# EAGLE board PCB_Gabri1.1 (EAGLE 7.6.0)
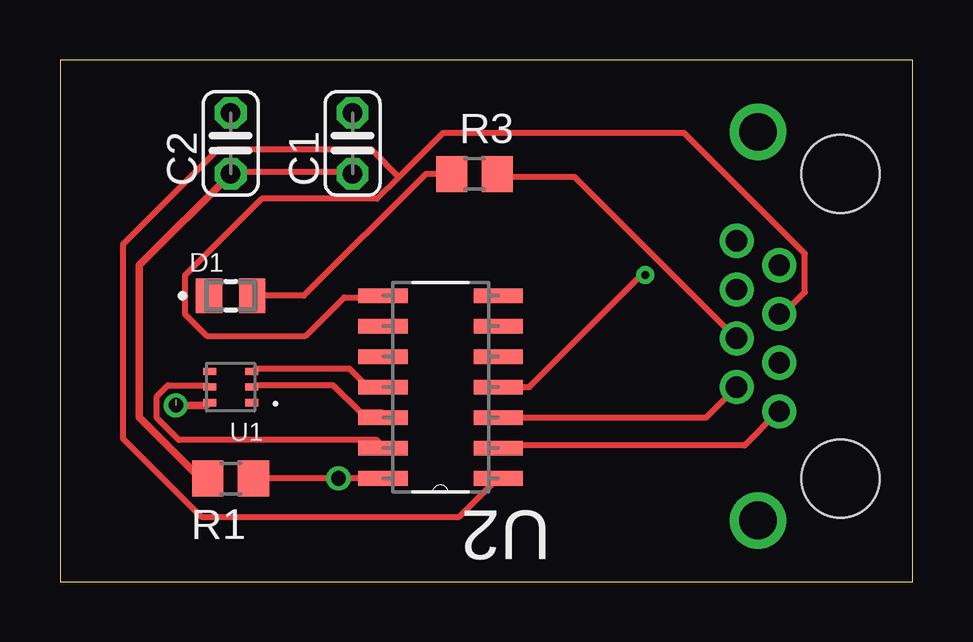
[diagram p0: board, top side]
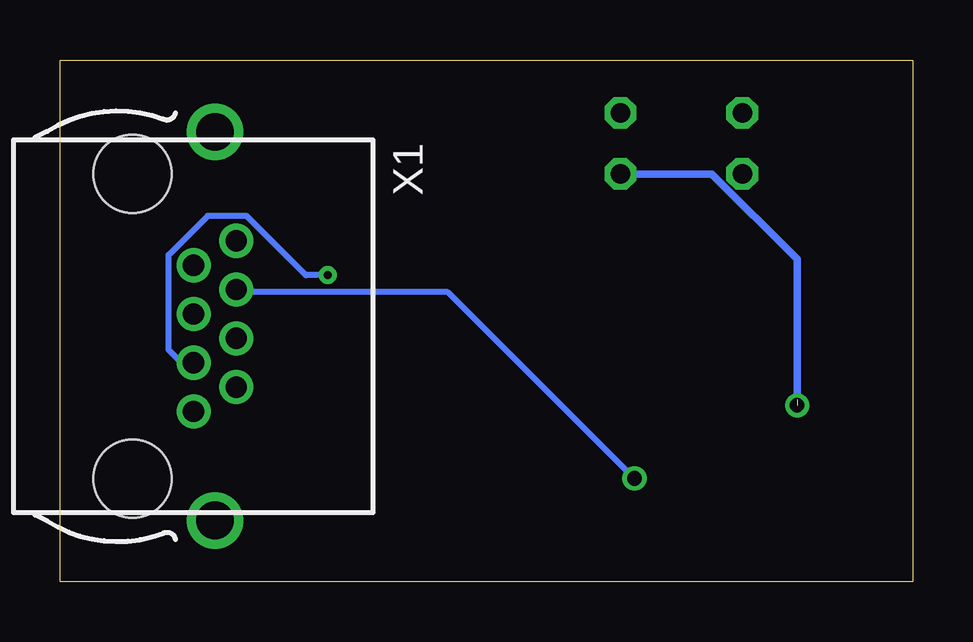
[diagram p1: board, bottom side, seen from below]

Size 35.54 x 21.77 mm. Coordinates in mm from the lower left corner, seen from the top.
Outline: 0,0 35.54,0 35.54,21.77 0,21.77 0,0
Copper layers (1*16): Top 0.035mm / dielectric 1.5mm / Bottom 0.035mm
Design rules "default": minimum track width 10mil, minimum drill 24mil, track to track 8mil, track to pad 8mil, pad to pad 8mil, via to via 8mil, smd to smd 8mil, copper to edge 40mil, drill to drill 8mil, minimum pad ring 10mil, minimum via ring 8mil, stop-mask expansion 4mil, vias tented up to drill 0mil, thermal gap 10mil
tRestrict: area 14,4.1 to 17.5,12.2; 8 lines

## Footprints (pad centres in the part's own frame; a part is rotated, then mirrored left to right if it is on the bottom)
C025-024X044 = drill 0.813 octagon: 1 -1.27,0; 2 1.27,0
LEDC2012X70N = smd 1.1 x 1.45: A 0.9,0; C -0.9,0
R0805 = smd 1.3 x 1.5: 1 -0.95,0; 2 0.95,0
VISHAY_VEML6030_2X2X0.87 = smd 0.55 x 0.3: 1 -0.875,0.65; 2 -0.875,0; 3 -0.875,-0.65; 4 0.875,-0.65; 5 0.875,0; 6 0.875,0.65
SOIC127P600X175-14N = smd 2.057 x 0.61: 1 -4.801,7.62; 2 -4.801,6.35; 3 -4.801,5.08; 4 -4.801,3.81; 5 -4.801,2.54; 6 -4.801,1.27; 7 -4.801,0; 8 0,0; 9 0,1.27; 10 0,2.54; 11 0,3.81; 12 0,5.08; 13 0,6.35; 14 0,7.62
0446200002 = drill 0.889 pad 1.422: 1 3.556,2.54; 2 2.54,4.318; 3 1.524,2.54; 4 0.508,4.318; 5 -0.508,2.54; 6 -1.524,4.318; 7 -2.54,2.54; 8 -3.556,4.318 | drill 1.575 pad 2.286: S@1 -8.103,3.429; S@2 8.103,3.429 | hole 3.251: 6.35,0; -6.35,0

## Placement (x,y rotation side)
C1  [C025-024X044]  12.19,18.29 90 top
C2  [C025-024X044]  7.11,18.29 90 top
D1  5988170107F  [LEDC2012X70N]  7.11,11.94 0 top
R1  [R0805]  7.11,4.32 180 top
R3  [R0805]  17.27,17.02 0 top
U1  VEML6030  [VISHAY_VEML6030_2X2X0.87]  7.11,8.13 180 top
U2  TXS0104ED  [SOIC127P600X175-14N]  13.46,11.94 180 top
X1  0446200002  [0446200002]  32.51,10.67 270 bottom

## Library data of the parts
C1 C2 R1 R3 = resistor
D1 = 5988170107F; AVAILABILITY: Unavailable; DESCRIPTION: LED GREEN CLEAR 0805 SMD; MF: Dialight; MP: 5988170107F; PACKAGE: 0805 Dialight; PRICE: None
U1 = VEML6030; AVAILABILITY: Unavailable; DESCRIPTION: VEML6030 Series 2 x 2 x 0.85 mm 50 mW I2C High Accuracy Ambient Light Sensor; MF: Vishay; MP: VEML6030; PACKAGE: SMD-6 Vishay; PRICE: None
U2 = TXS0104ED; AVAILABILITY: Unavailable; DESCRIPTION: 4-Bit Bidirectional Voltage-Level Shifter for Open-Drain and Push-Pull Applications 14-SOIC -40 to 85; MF: Texas Instruments; MP: TXS0104ED; PACKAGE: SOIC-14 Texas Instruments; PRICE: None
X1 = 0446200002; AVAILABILITY: Unavailable; DESCRIPTION: Conn RJ-45 RCP 8 POS 2.04mm Solder RA Thru-Hole 8 Terminal 1 Port Tray Cat 3; MF: Molex, LLC; MP: 0446200002; PACKAGE: None; PRICE: None

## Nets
A1: U2.2 X1.1
A2: U2.3 X1.2
A3: U2.4 X1.3
GND: U1.1
INT: U1.3 U2.11
LED_1: R3.2 X1.4
LED_2: D1.A R3.1
LS_VDD: C1.1 C2.1
N$1: R1.2
S$1: U1.6
SCL: U1.5 U2.13
SDA: U1.2 U2.12
VCCA: U2.1 U2.8 X1.5
VCCB: R1.1 U2.14 X1.6

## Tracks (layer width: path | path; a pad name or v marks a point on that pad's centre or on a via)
A1
  Top 0.254: U2.2 18.47,5.69 28.52,5.69 29.9,7.06 X1.1
A2
  Top 0.254: U2.3 26.92,6.86 X1.2
A3  (via drill 0.35)
  Top 0.254: U2.4 19.56,8.13 24.23,12.8 v24.38,12.8
  Bottom 0.254: X1.3 30.48,9.14 31.01,9.68 31.01,13.64 29.39,15.26 27.76,15.26 25.3,12.8 v24.38,12.8
INT
  Top 0.254: U1.3 8.18,8.89 12.06,8.89 12.75,8.2 13.44,8.2 U2.11
LED_1
  Top 0.254: R3.2 18.24,16.89 21.44,16.89 28.07,10.26 X1.4
LED_2
  Top 0.254: R3.1 15.24,17.02 10.16,11.94 D1.A
LS_VDD  (via drill 0.6)  (1 unrouted)
  Top 0.254: C1.1 12.06,17.12 7.26,17.12 C2.1 7.29,17.15
  Top 0.305: 5.59,4.57 3.3,6.86 3.3,13.21 C2.1 | 6.1,7.37 v4.83,7.37
  Bottom 0.305: C1.1 8.38,17.02 4.83,13.46 v4.83,7.37
N$1
  Top 0.254: 6.12,4.32 R1.2
S$1
  Top 0.254: 6.12,7.52 U1.6
SCL
  Top 0.254: U1.5 6.12,8.2 4.5,8.2 4.04,7.75 4.04,6.83 4.95,5.92 13.21,5.92 13.44,5.69 U2.13
SDA
  Top 0.254: U1.2 8.18,8.2 11.38,8.2 12.52,7.06 13.44,7.06 U2.12
VCCA
  Top 0.254: 14.12,16.89 15.95,18.72 26.01,18.72 31.04,13.69 31.04,12.09 30.12,11.18 X1.5 | 14.12,16.89 13.21,15.98 8.41,15.98 5.21,12.78 5.21,11.18 6.12,10.26 10.24,10.26 11.84,11.86 13.44,11.86 U2.8 | 14.12,16.89 12.98,18.03 6.58,18.03 2.62,14.07 2.62,5.99 5.89,2.72 16.64,2.72 18.24,4.32 U2.1
VCCB  (via drill 0.61)
  Top 0.254: U2.14 v11.61,4.32 R1.1
  Bottom 0.254: v11.61,4.32 19.38,12.09 28.07,12.09 X1.6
